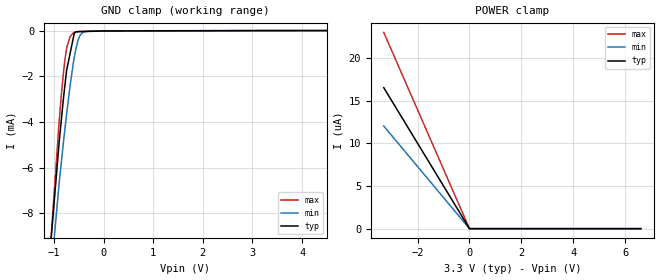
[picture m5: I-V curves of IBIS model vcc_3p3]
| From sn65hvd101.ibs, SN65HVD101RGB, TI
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|   vcc_3p3 Model
[Model]   vcc_3p3
Model_type   Input
Vinl = 0.8
Vinh = 2.0
|   typ   min   max
|   (nom PVT)   (fast PVT)   (slow PVT)
C_comp   8.028e-13   7.642e-13   8.321e-13
| Where nom  PVT is Nominal Process, 3.3V, 45C
|   Fast PVT is Strong Process,  3.6V, -20C
|   Slow PVT is Weak Process,   3V, 125C
[Voltage Range]   3.3   3   3.6
|Junction Temperature
[Temperature Range]   45   125   -20
[Power Clamp Reference]   3.3   3   3.6
[GND Clamp Reference]   0   0   0
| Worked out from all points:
|   GND clamp passes 1 mA (typ) near -0.67 V on its own axis
[GND Clamp]
|   Voltage   I(typ)   I(min)   I(max)
-3.3V     -95.24mA   -81.22mA   -114.6mA
-1.127V   -10.94mA   -12.29mA   -11.21mA
-897.6mV  -4.95mA    -6.735mA   -4.038mA
-813.6mV  -3.074mA   -4.981mA   -1.955mA
-777.6mV  -2.372mA   -4.285mA   -1.261mA
-745.8mV  -1.752mA   -3.672mA   -800.5uA
-676.8mV  -1.026mA   -2.459mA   -280.7uA
-590.7mV  -119.5uA   -1.183mA   -77.61uA
-572.4mV  -84.69uA   -968.2uA   -57.3uA
-471mV    -46.89uA   -193.2uA   -35.54uA
-285mV    -34.82uA   -13.78uA   -27.22uA
6.6V      0A         0A         0A
[POWER Clamp]
|   Voltage   I(typ)   I(min)   I(max)
-3.3V     16.54uA    12.04uA    23.02uA
-60mV     300.8nA    219.5nA    418.6nA
-33.83fV  0A         0A         0A
6.6V      0A         0A         0A
